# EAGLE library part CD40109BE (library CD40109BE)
CD40109BE, Voltage Level Shifter 3-State 3 18 V 16-Pin PDIP Source: Datasheet
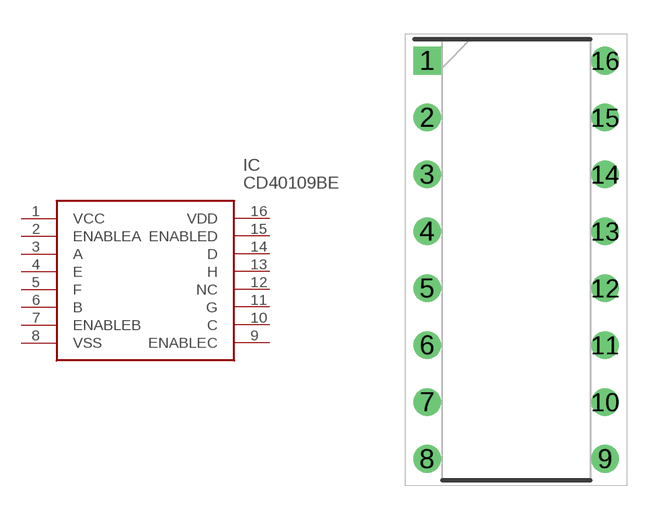
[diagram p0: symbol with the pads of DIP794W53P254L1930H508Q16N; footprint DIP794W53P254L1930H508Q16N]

Designator prefix IC

## CD40109BE (Arrow_Part_Number: CD40109BE; Arrow_Price-Stock: https://www.arrow.com/en/products/cd40109be/texas-instruments?utm_currency=USD&region=nac; Description: CD40109BE, Voltage Level Shifter 3-State 3 18 V 16-Pin PDIP; Height: 5.08mm; Manufacturer_Name: Texas Instruments; Manufacturer_Part_Number: CD40109BE; Mouser_Part_Number: 595-CD40109BE; Mouser_Price-Stock: https://www.mouser.co.uk/ProductDetail/Texas-Instruments/CD40109BE?qs=gb35HGp1gQIrpwwQZIZgDQ%3D%3D)  [DIP794W53P254L1930H508Q16N]
1  VCC  pwr
2  ENABLEA
3  A
4  E
5  F
6  B
7  ENABLEB
8  VSS  pwr
9  ENABLEC
10  C
11  G
12  NC  nc
13  H
14  D
15  ENABLED
16  VDD  pwr

## Footprint DIP794W53P254L1930H508Q16N (pad centres in mm)
N (R-PDIP-T16)
drill 0.73 pad 1.13 square: 1 -3.97,8.89
drill 0.73 pad 1.13: 2 -3.97,6.35; 3 -3.97,3.81; 4 -3.97,1.27; 5 -3.97,-1.27; 6 -3.97,-3.81; 7 -3.97,-6.35; 8 -3.97,-8.89; 9 3.97,-8.89; 10 3.97,-6.35; 11 3.97,-3.81; 12 3.97,-1.27; 13 3.97,1.27; 14 3.97,3.81; 15 3.97,6.35; 16 3.97,8.89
